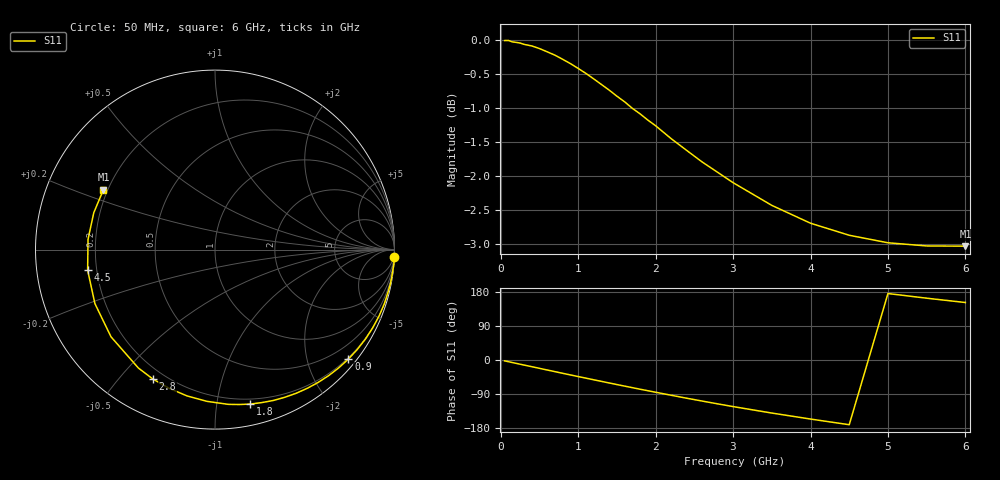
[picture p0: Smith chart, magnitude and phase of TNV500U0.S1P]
! SIEMENS Discrete & RF Semiconductors
! BAS70-07W
! Si Schottky Diode in SOT343
! VR = 0.5 V
! S-Parameters:  February  1997
# GHz  S  MA  R  50
!  f  S11
! GHz  MAG  ANG
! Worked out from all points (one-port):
!   34 points, 50 MHz to 6 GHz, reference 50 ohm
!   lowest |S11| = -3.0 dB at 6 GHz (marker M1), VSWR 5.80, Z = 9.16 + j12.2 ohm
!   |S11| at or under -10 dB: nowhere
!   S11 on the Smith chart (normalised r, x): 50 MHz: 0, -50; 900 MHz: 0.17, -2.78; 1.8 GHz: 0.16, -1.24; 2.8 GHz: 0.15, -0.62; 4.5 GHz: 0.16, -0.08; 6 GHz: 0.18, +0.24
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0.05  0.9997 -2.3
0.1  0.9999 -4.5
0.25  0.9955 -11.1
0.4  0.9907 -17.6
0.5  0.9863 -22.0
0.6  0.9808 -26.4
0.7  0.9753 -30.7
0.8  0.9684 -35.1
0.9  0.9614 -39.4
1  0.9536 -43.7
1.2  0.9369 -52.2
1.3  0.9281 -56.4
1.4  0.9192 -60.6
1.5  0.9098 -64.8
1.6  0.9011 -68.9
1.8  0.8829 -77.1
2  0.8653 -85.1
2.2  0.8467 -93.0
2.4  0.83 -100.8
2.6  0.8139 -108.3
2.8  0.7998 -115.7
3  0.7858 -122.9
3.5  0.7562 -140.0
4  0.7337 -155.8
4.5  0.7188 -170.8
5  0.7097 175.4
5.5  0.7059 163.1
6  0.7057 151.7
